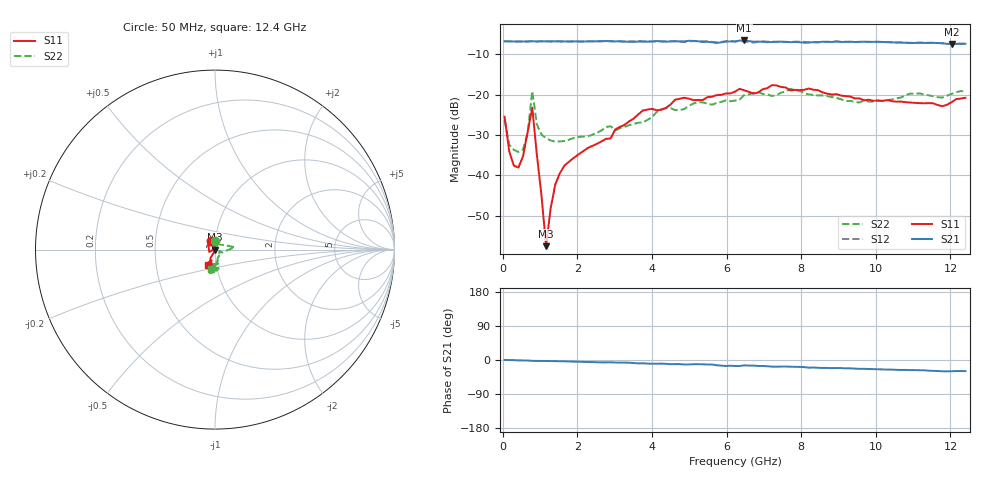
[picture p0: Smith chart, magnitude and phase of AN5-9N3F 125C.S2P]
! Network Analyzer HP8720D.06.14 Serial No. US36140669
! 24 Jul 2008  15:15:34
! Frequency  S11  S21  S12  S22
# HZ  S  DB R 50
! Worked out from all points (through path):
!   101 points, 50 MHz to 12.4 GHz, reference 50 ohm
!   highest |S21| = -6.54 dB at 6.472 GHz (marker M1); lowest = -7.4 dB at 12.03 GHz (marker M2)
!   group delay of S21, straight-line fit = 6.85 ps
!   lowest |S11| = -57.5 dB at 1.161 GHz (marker M3), VSWR 1.00, Z = 49.9 + j0.0515 ohm
!   |S11| at or under -10 dB: start of sweep to end of sweep
!   |S22| runs from -34.2 to -18.5 dB; largest |S21 - S12| = 0.014
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5e7  -25.46 116.7  -6.74 0.2  -6.78 0.1  -26.22 90.2
1.735e8  -34.03 129.0  -6.75 -0.1  -6.77 -0.3  -32.40 61.5
2.97e8  -37.56 148.7  -6.79 -0.3  -6.78 -0.5  -33.67 52.5
4.205e8  -38.06 174.4  -6.80 -0.9  -6.78 -1.0  -34.19 51.4
5.44e8  -35.27 -163.3  -6.79 -1.2  -6.78 -1.2  -33.59 59.7
6.675e8  -29.27 -157.1  -6.79 -1.4  -6.79 -1.4  -29.49 77.9
7.91e8  -23.21 128.2  -6.73 -2.2  -6.73 -2.2  -19.10 7.2
9.145e8  -34.84 88.8  -6.79 -2.4  -6.78 -2.3  -27.36 -22.9
1.1615e9  -57.54 157.1  -6.76 -2.6  -6.77 -2.5  -30.74 -17.3
1.285e9  -48.02 -130.4  -6.77 -2.9  -6.79 -2.9  -31.35 -16.3
1.4085e9  -42.24 -121.1  -6.76 -3.1  -6.78 -3.2  -31.64 -18.5
1.6555e9  -37.55 -114.0  -6.79 -3.5  -6.78 -3.8  -31.48 -26.8
2.1495e9  -34.05 -113.1  -6.80 -5.0  -6.78 -4.9  -30.36 -36.3
3.755e9  -23.91 -113.2  -6.81 -8.7  -6.74 -8.2  -26.89 -67.6
4.249e9  -23.74 -110.7  -6.76 -9.5  -6.76 -9.8  -23.59 -71.4
4.6195e9  -21.23 -112.7  -6.72 -10.9  -6.77 -10.3  -23.82 -70.0
6.225e9  -19.25 -105.4  -6.81 -15.9  -6.77 -14.3  -21.45 -86.2
6.472e9  -18.90 -95.8  -6.54 -14.1  -6.80 -13.6  -20.08 -90.2
8.3245e9  -18.75 -96.2  -6.97 -19.8  -6.94 -19.5  -20.01 -81.4
1.0424e10  -21.59 -105.0  -7.00 -25.3  -6.99 -25.9  -21.19 -95.7
1.20295e10  -21.86 -106.8  -7.42 -29.7  -7.40 -29.7  -19.80 -97.9
1.24e10  -20.75 -113.8  -7.37 -29.3  -7.33 -29.3  -19.25 -102.3
